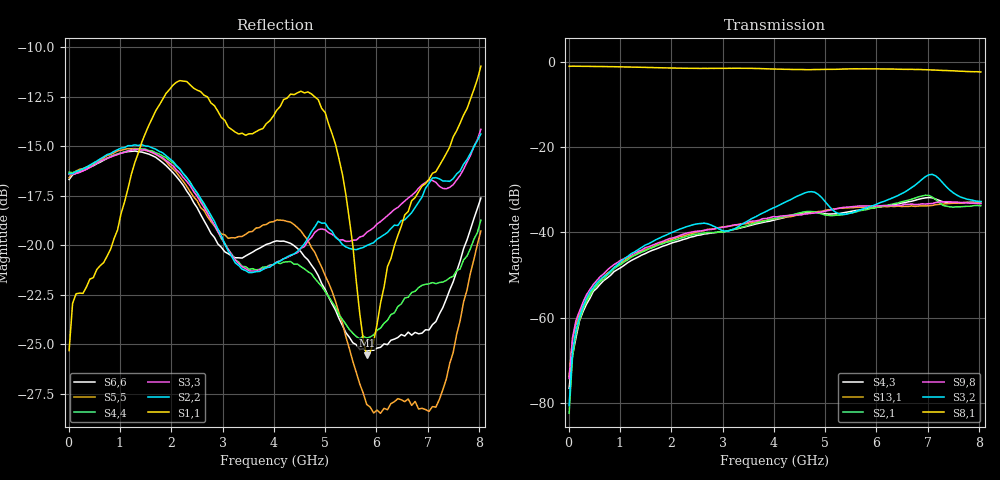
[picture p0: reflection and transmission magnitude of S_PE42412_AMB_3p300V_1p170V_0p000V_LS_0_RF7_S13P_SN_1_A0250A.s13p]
! Device ID: PE42412
! File Path: z:\PE42412\TE_GND_Post_Char_S-Param\All Parts\AMB\3p300\LS_0_RF7\PE42412_AMB_3p300V_1p170V_0p000V_LS_0_RF7_S13P_SN_1_A0250A.s13p
! Serial: 1
! Lot: A0250A
! Temp: AMB
! VDD: 3.300
! VSS: 0.000
! Control_Hi: 1.170
! Control_Lo: 0.000
! Logic State: LS_0_RF7
! Port 1:
! Port 2:
! Port 3:
! Port 4:
! Port 5:
! Port 6:
! Port 7:
! Port 8:
! Port 9:
! Port 10:
! Port 11:
! Port 12:
! Port 13:
! ThroughPath:1-8
! IDD: 0.0001071059
! ISS/IDD2: -3.1e-008
! IDMM3/IDD3: -1.926e-007
! Comment:
#  Hz  S  RI  R  50
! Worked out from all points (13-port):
!   120 points, 10 MHz to 8.037 GHz, reference 50 ohm
!   strongest paths, dB at 10 MHz, 2.034 GHz, 4.057 GHz, 6.08 GHz, 8.037 GHz:
!     S8,1: -1.0, -1.4, -1.7, -1.6, -2.3
!     S3,2: -80.7, -39.9, -33.9, -33.0, -32.7
!     S9,8: -74.3, -41.3, -36.4, -33.8, -33.2
!     S2,1: -82.5, -42.0, -36.7, -34.0, -33.7
!     S13,1: -73.8, -41.6, -36.8, -34.0, -33.2
!     S4,3: -76.6, -42.4, -37.0, -34.0, -32.8
!   lowest |S11| = -25.6 dB at 5.811 GHz (marker M1), VSWR 1.11, Z = 54.9 + j2.5 ohm
!   |S11| at or under -10 dB: start of sweep to end of sweep
